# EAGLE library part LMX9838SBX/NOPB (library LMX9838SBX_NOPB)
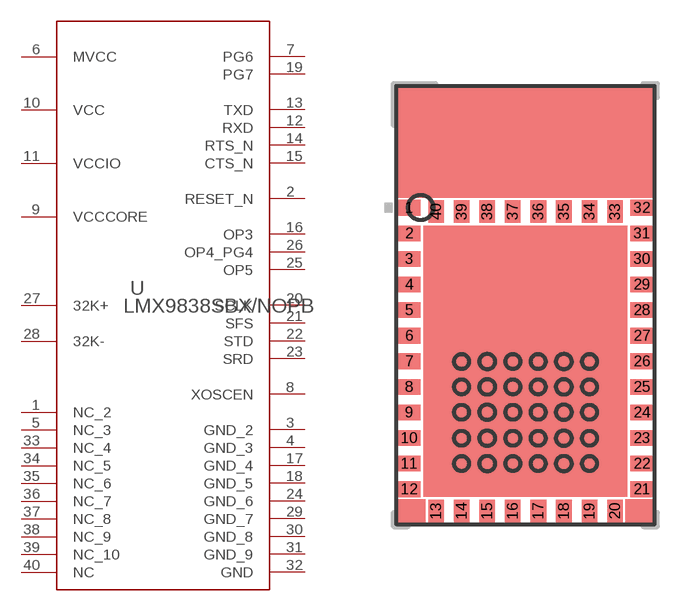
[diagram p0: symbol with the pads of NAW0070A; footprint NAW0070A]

Designator prefix U

## LMX9838SBX/NOPB (ALTERNATEPARTNUMBER: LMX9838SB/NOPB; APPLICATION_BUILDNUMBER: *; COMPTYPE: IC; MANUFACTURER: Texas Instruments; MOUNTTYPE: SMT; PACKAGEREFERENCE: NAW0070A; PARTNUMBER: LMX9838SBX/NOPB; PIN_COUNT: 40; REFDES: RefDes; ROHS: Y; TYPE: TYPE; VALUE: Value)  [NAW0070A]
1  NC_2  pas
2  RESET_N  in
3  GND_2  pwr
4  GND_3  pwr
5  NC_3  pas
6  MVCC  pwr
7  PG6
8  XOSCEN  out
9  VCCCORE  pwr
10  VCC  pwr
11  VCCIO  pwr
12  RXD  in
13  TXD  out
14  RTS_N  out
15  CTS_N  in
16  OP3  in
17  GND_4  pwr
18  GND_5  pwr
19  PG7
20  SCLK
21  SFS
22  STD  out
23  SRD  in
24  GND_6  pwr
25  OP5
26  OP4_PG4
27  32K+  in
28  32K-  out
29  GND_7  pwr
30  GND_8  pwr
31  GND_9  pwr
32  GND  pwr
33  NC_4  pas
34  NC_5  pas
35  NC_6  pas
36  NC_7  pas
37  NC_8  pas
38  NC_9  pas
39  NC_10  pas
40  NC  pas

## Footprint NAW0070A (pad centres in mm)
smd 0.889 x 0.61: 1 -4.55,3.8; 2 -4.55,2.8; 3 -4.55,1.8; 4 -4.55,0.8; 5 -4.55,-0.2; 6 -4.55,-1.2; 7 -4.55,-2.2; 8 -4.55,-3.2; 9 -4.55,-4.2; 10 -4.55,-5.2; 11 -4.55,-6.2; 12 -4.55,-7.2; 21 4.55,-7.2; 22 4.55,-6.2; 23 4.55,-5.2; 24 4.55,-4.2; 25 4.55,-3.2; 26 4.55,-2.2; 27 4.55,-1.2; 28 4.55,-0.2; 29 4.55,0.8; 30 4.55,1.8; 31 4.55,2.8; 32 4.55,3.8
smd 0.61 x 0.889: 13 -3.5,-8.05; 14 -2.5,-8.05; 15 -1.5,-8.05; 16 -0.5,-8.05; 17 0.5,-8.05; 18 1.5,-8.05; 19 2.5,-8.05; 20 3.5,-8.05; 33 3.5,3.65; 34 2.5,3.65; 35 1.5,3.65; 36 0.5,3.65; 37 -0.5,3.65; 38 -1.5,3.65; 39 -2.5,3.65; 40 -3.5,3.65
